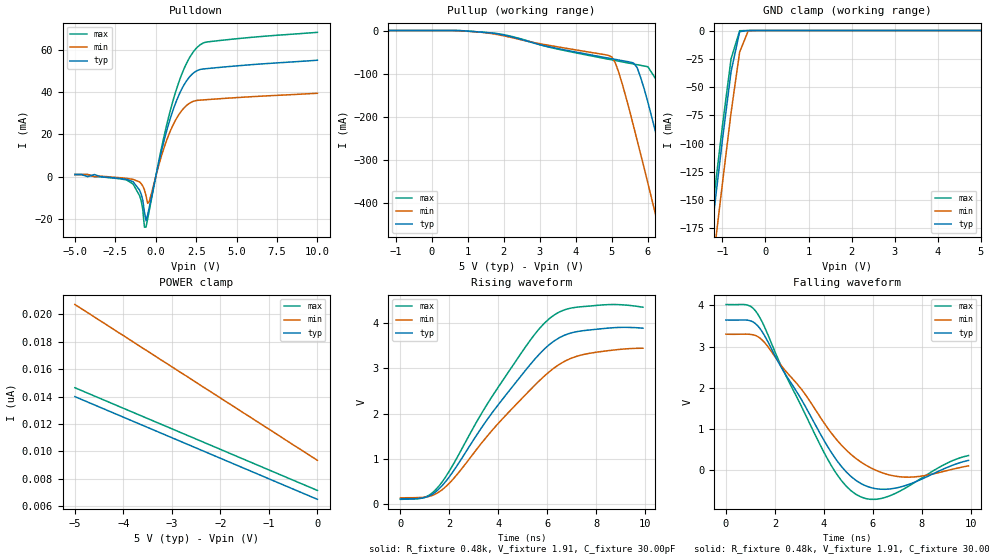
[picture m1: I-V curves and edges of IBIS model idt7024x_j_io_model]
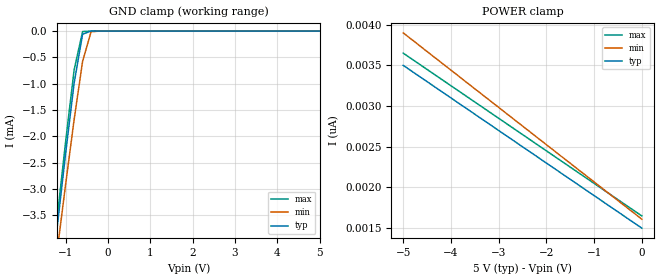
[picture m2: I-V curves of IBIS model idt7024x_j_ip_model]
| IBIS file 7024j.ibs created by s2ibis2 version 1.0
| North Carolina State University Electronics Research Laboratory  1995
[IBIS ver]   2.1
[File name]   7024j.ibs
[File Rev]   3.1
[Date]   06/13/97
[Source]   Integrated Device Technology, Inc.
[Notes]   1.Temperatures: typ=25C, min=100C, max=0C 2.Cemos7_5v process.
   3.RRmp rates based on 50 ohm load.
[Disclaimer]   This information is for modeling purpose only, and is not
   guaranteed.
[Copyright]   Copyright 1997, Integrated Device Technology, Inc. all rights
   reserved
|   Component idt7024x_j
[Component]   7024j
[Manufacturer]   Integrated Device Technology
[Package]
| variable   typ   min   max
R_pkg   100.00m   50.00m   0.15
L_pkg   12.00nH   11.00nH   13.00nH
C_pkg   0.80pF   0.70pF   0.90pF
[Pin]  signal_name   model_name   R_pin   L_pin   C_pin
1   VCC   POWER
2   OEBL   idt7024x_j_ip_model
3   IO0L   idt7024x_j_io_model
4   IO1L   idt7024x_j_io_model
5   GND   GND
6   IO2L   idt7024x_j_io_model
7   IO3L   idt7024x_j_io_model
8   IO4L   idt7024x_j_io_model
9   IO5L   idt7024x_j_io_model
10   IO6L   idt7024x_j_io_model
11   IO7L   idt7024x_j_io_model
12   IO8L   idt7024x_j_io_model
13   IO9L   idt7024x_j_io_model
14   IO10L   idt7024x_j_io_model
15   IO11L   idt7024x_j_io_model
16   IO12L   idt7024x_j_io_model
17   IO13L   idt7024x_j_io_model
18   GND   GND
19   IO14L   idt7024x_j_io_model
20   IO15L   idt7024x_j_io_model
21   VCC   POWER
22   GND   GND
23   IO0R   idt7024x_j_io_model
24   IO1R   idt7024x_j_io_model
25   IO2R   idt7024x_j_io_model
26   VCC   POWER
27   IO3R   idt7024x_j_io_model
28   IO4R   idt7024x_j_io_model
29   IO5R   idt7024x_j_io_model
30   IO6R   idt7024x_j_io_model
31   IO7R   idt7024x_j_io_model
32   IO8R   idt7024x_j_io_model
33   IO9R   idt7024x_j_io_model
34   IO10R   idt7024x_j_io_model
35   IO11R   idt7024x_j_io_model
36   IO12R   idt7024x_j_io_model
37   IO13R   idt7024x_j_io_model
38   IO14R   idt7024x_j_io_model
39   GND   GND
40   IO15R   idt7024x_j_io_model
41   OEBR   idt7024x_j_ip_model
42   RWBR   idt7024x_j_ip_model
43   GND   GND
44   SEMBR   idt7024x_j_ip_model
45   CEBR   idt7024x_j_ip_model
46   UBR   idt7024x_j_ip_model
47   LBR   idt7024x_j_ip_model
48   NC   NC
49   A11R   idt7024x_j_ip_model
50   A10R   idt7024x_j_ip_model
51   A9R   idt7024x_j_ip_model
52   A8R   idt7024x_j_ip_model
53   A7R   idt7024x_j_ip_model
54   A6R   idt7024x_j_ip_model
55   A5R   idt7024x_j_ip_model
56   A4R   idt7024x_j_ip_model
57   A3R   idt7024x_j_ip_model
58   A2R   idt7024x_j_ip_model
59   A1R   idt7024x_j_ip_model
60   A0R   idt7024x_j_ip_model
61   INTBR   idt7024x_j_ip_model
62   BUSYBR   idt7024x_j_io_model
63   MSBR   idt7024x_j_ip_model
64   GND   GND
65   BUSYBL   idt7024x_j_io_model
66   INTBL   idt7024x_j_ip_model
67   A0L   idt7024x_j_ip_model
68   A1L   idt7024x_j_ip_model
69   A2L   idt7024x_j_ip_model
70   A3L   idt7024x_j_ip_model
71   A4L   idt7024x_j_ip_model
72   A5L   idt7024x_j_ip_model
73   A6L   idt7024x_j_ip_model
74   A7L   idt7024x_j_ip_model
75   A8L   idt7024x_j_ip_model
76   A9L   idt7024x_j_ip_model
77   A10L   idt7024x_j_ip_model
78   A11L   idt7024x_j_ip_model
79   NC   NC
80   LBL   idt7024x_j_ip_model
81   UBL   idt7024x_j_ip_model
82   CEBL   idt7024x_j_ip_model
83   SEMBL   idt7024x_j_ip_model
84   RWBL   idt7024x_j_ip_model
| Models and submodels in the file (2): idt7024x_j_io_model (I/O), idt7024x_j_ip_model (Input)
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| in   in   dummy_model
| oel  oel   dummy_model
|   Model idt7024x_j_io_model
[Model]   idt7024x_j_io_model
Model_type   I/O
Polarity   Non-Inverting
Enable   Active-High
Vinl =  0.800V
Vinh =  2.200V
Vmeas =  1.500V
C_comp   3.00pF   NA   NA
[Temperature Range]   25.00   100.00   0.000
[Voltage Range]   5.00V   4.50V   5.50V
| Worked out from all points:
|   slope of the pulldown table from 0 to 0.75 V, typ, clamps not added: 31.6 ohm
|   slope of the pullup table from 0 to 0.75 V, typ, clamps not added: 3.95 kohm
|   GND clamp passes 1 mA (typ) near -0.60 V on its own axis
|   rising waveform, R_fixture 0.48k, V_fixture 1.91, C_fixture 30.00pF: 20-80 % time 3.04ns typ, 3.26ns min, 2.91ns max; typ from 0.106 V to 3.89 V
|   falling waveform, R_fixture 0.48k, V_fixture 1.91, C_fixture 30.00pF: 20-80 % time 1.97ns typ, 2.4ns min, 1.74ns max; typ from 3.64 V to 0.242 V
[Pulldown]
| voltage   I(typ)   I(min)   I(max)
-5V       1mA        1mA        1mA
-1.4V     -2.4mA     -1.3mA     -3.5mA
-900mV    -8.3mA     -3.3mA     -11.35mA
-700mV    -16.78mA   -6.19mA    -23.89mA
-600mV    -20.9mA    -9.09mA    -23.8mA
-400mV    -14.53mA   -11.73mA   -16.03mA
400mV     13.58mA    10.94mA    15.15mA
1V        29.9mA     23.3mA     34.1mA
1.7V      42.75mA    32.09mA    50.15mA
2.5V      49.92mA    36.01mA    60.67mA
3.2V      51.14mA    36.46mA    63.76mA
10V       55.08mA    39.44mA    68.28mA
[Pullup]
| voltage   I(typ)   I(min)   I(max)
-5V       -500pA     -450pA     -550pA
1.5V      -4.551mA   -5.174mA   -4.555mA
4.9V      -63.93mA   -57.43mA   -66.49mA
5.1V      -66.99mA   -75.6mA    -69.7mA
5.6V      -75.23mA   -221mA     -77.66mA
5.7V      -85.71mA   -254mA     -79.24mA
6V        -166mA     -354mA     -83.98mA
6.4V      -296mA     -491mA     -136mA
6.8V      -433mA     -628mA     -260mA
7.2V      -571mA     -766mA     -396mA
7.6V      -710mA     -905mA     -534mA
10V       -1.549A    -1.74A     -1.373A
[GND_clamp]
| voltage   I(typ)   I(min)   I(max)
-5V       -1.454A    -1.488A    -1.443A
-1.4V     -227mA     -265mA     -214mA
-1.2V     -161mA     -199mA     -148mA
-1V       -96.53mA   -135mA     -84.09mA
-800mV    -36.33mA   -72.6mA    -25.03mA
-600mV    -974uA     -19.01mA   -145uA
-400mV    -381nA     -207uA     -24.45nA
5V        6.5nA      10.48nA    6.399nA
[POWER_clamp]
| voltage   I(typ)   I(min)   I(max)
-5V       14nA       20.73nA    14.65nA
-1V       7.998nA    11.63nA    8.648nA
-500mV    7.248nA    10.48nA    7.898nA
0V        6.5nA      9.346nA    7.148nA
[Ramp]
| variable   typ   min   max
dV/dt_r   1.09/2.35n   0.91/2.40n   1.25/2.28n
dV/dt_f   1.50/1.81n   1.08/1.74n   1.81/1.81n
R_load = 50.00
[Rising Waveform]
R_fixture = 0.48k
V_fixture = 1.91
C_fixture = 30.00pF
R_dut = 100.00m
L_dut = 12.00nH
C_dut = 0.80pF
| time   V(typ)   V(min)   V(max)
0s        106mV      128mV      96.44mV
1ns       137mV      146mV      142mV
1.6ns     343mV      270mV      409mV
2.2ns     754mV      576mV      913mV
3.8ns     2.058V     1.663V     2.428V
5.3ns     3.089V     2.527V     3.627V
6.1ns     3.539V     2.938V     4.116V
6.7ns     3.739V     3.159V     4.302V
7.4ns     3.835V     3.301V     4.371V
9.9ns     3.894V     3.45V      4.36V
[Falling Waveform]
R_fixture = 0.48k
V_fixture = 1.91
C_fixture = 30.00pF
R_dut = 100.00m
L_dut = 12.00nH
C_dut = 0.80pF
| time   V(typ)   V(min)   V(max)
0s        3.644V     3.3V       4.02V
900ps     3.639V     3.3V       4.001V
1.3ns     3.501V     3.241V     3.786V
3.1ns     1.696V     1.952V     1.525V
4.1ns     627mV      1.068V     325mV
4.7ns     104mV      619mV      -237mV
5.3ns     -241mV     291mV      -579mV
6.2ns     -450mV     -18.43mV   -695mV
7.3ns     -372mV     -164mV     -437mV
9.9ns     242mV      109mV      359mV
|   Model idt7024x_j_ip_model
[Model]   idt7024x_j_ip_model
Model_type   Input
Vinl =  0.800V
Vinh =  2.200V
Vmeas =  1.500V
C_comp   3.00pF   NA   NA
[Temperature Range]   25.00   100.00   0.000
[Voltage Range]   5.00V   4.50V   5.50V
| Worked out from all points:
|   GND clamp passes 1 mA (typ) near -0.80 V on its own axis
[GND_clamp]
| voltage   I(typ)   I(min)   I(max)
-5V       -31.79mA   -29.37mA   -32.66mA
-1.4V     -5.161mA   -5.465mA   -5.039mA
-1.2V     -3.726mA   -4.176mA   -3.551mA
-1V       -2.319mA   -2.908mA   -2.095mA
-800mV    -988uA     -1.682mA   -736uA
-600mV    -59.14uA   -575uA     -8.563uA
-400mV    -28.28nA   -13.79uA   -2.35nA
-200mV    -591pA     -29.53nA   -630pA
5V        1.5nA      1.839nA    1.45nA
[POWER_clamp]
| voltage   I(typ)   I(min)   I(max)
-5V       3.5nA      3.899nA    3.65nA
-1.7V     2.18nA     2.388nA    2.33nA
-1.2V     1.98nA     2.16nA     2.13nA
0V        1.5nA      1.61nA     1.65nA
